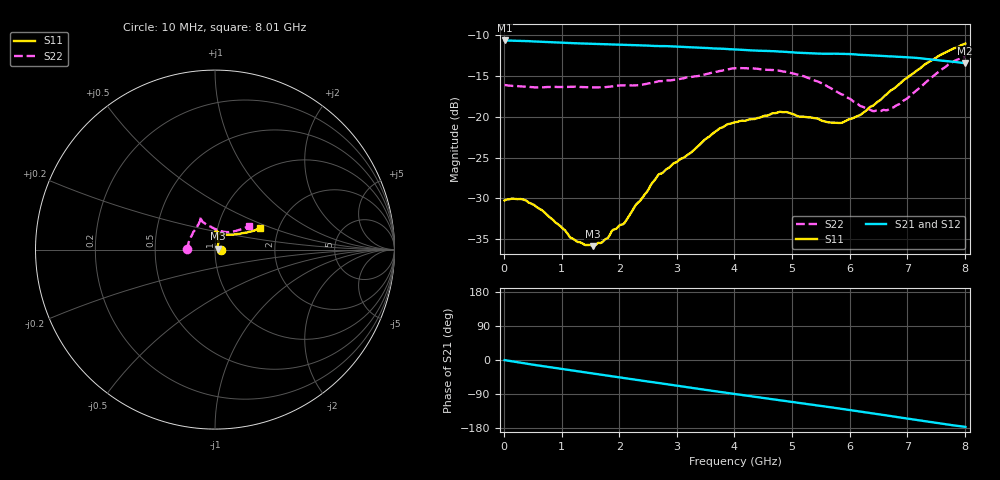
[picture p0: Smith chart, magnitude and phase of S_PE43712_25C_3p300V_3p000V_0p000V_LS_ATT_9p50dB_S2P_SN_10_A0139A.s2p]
! DEVICE ID: PE43712
! File Path: z:\PE43713\PE43713_CHAR_NOM_04292014\AMB\3p300\LS_ATT_9p50dB\PE43713_AMB_3p300V_3p000V_0p000V_LS_ATT_9p50dB_S2P_SN_10_A0139A.s2p
! Serial: 10
! Lot: A0139A
! Temp: 25C
! VDD: 3.300
! VSS: 0.000
! Control_Hi: 3.000
! Control_Lo: 0.000
! Attenuation Step: 9.50dB
! Port 1: RF1
! Port 2: RF2
! ThroughPath:1-2
! IDD: 0.0001469591
! ISS: -2.49e-008
#  Hz  S  RI  R  50
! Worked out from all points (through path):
!   801 points, 10 MHz to 8.01 GHz, reference 50 ohm
!   highest |S21| = -10.66 dB at 10 MHz (marker M1); lowest = -13.4 dB at 8 GHz (marker M2)
!   group delay of S21, straight-line fit = 60.6 ps
!   lowest |S11| = -35.9 dB at 1.54 GHz (marker M3), VSWR 1.03, Z = 51.6 + j0.514 ohm
!   |S11| at or under -10 dB: start of sweep to end of sweep
!   |S22| runs from -19.3 to -12.7 dB; largest |S21 - S12| = 0.0011
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1e7  0.0307 0.000143  0.2932 -0.00153  0.2933 -0.00148  -0.1564 0.000949
3e8  0.0311 -0.00359  0.2886 -0.0381  0.2886 -0.0381  -0.1526 0.0151
5e8  0.0287 -0.0048  0.2827 -0.0616  0.2827 -0.0616  -0.1498 0.0238
1.17e9  0.0181 -0.000596  0.2505 -0.1303  0.2505 -0.1305  -0.1422 0.0552
1.35e9  0.0168 0.00151  0.2398 -0.1467  0.2398 -0.1467  -0.1386 0.0623
1.54e9  0.0153 0.00498  0.2273 -0.1629  0.2273 -0.1629  -0.133 0.0717
1.71e9  0.0147 0.00871  0.2154 -0.1765  0.2154 -0.1765  -0.1289 0.0795
2.09e9  0.0139 0.0175  0.1857 -0.2041  0.1857 -0.204  -0.1211 0.0977
2.68e9  0.0192 0.0397  0.1329 -0.2361  0.1328 -0.2361  -0.0985 0.1322
3.72e9  0.0136 0.0826  0.0297 -0.2596  0.0295 -0.2596  -0.0825 0.1707
4.01e9  0.0104 0.0919  0.000998 -0.2584  0.000956 -0.2584  -0.085 0.179
4.79e9  0.00542 0.1071  -0.0707 -0.2404  -0.0708 -0.2407  -0.0802 0.1734
5.35e9  0.0159 0.0971  -0.1152 -0.216  -0.1152 -0.2159  -0.0693 0.1549
5.88e9  0.0387 0.0837  -0.154 -0.1874  -0.1537 -0.1874  -0.0331 0.1323
6.18e9  0.0606 0.0824  -0.1727 -0.166  -0.1724 -0.166  -0.0045 0.1166
6.39e9  0.0805 0.0837  -0.1837 -0.1504  -0.1834 -0.1503  0.0172 0.1074
6.68e9  0.1128 0.0851  -0.1971 -0.1268  -0.1968 -0.1269  0.0508 0.0985
7e9  0.1476 0.0905  -0.2088 -0.0994  -0.2085 -0.0993  0.0846 0.098
7.35e9  0.1895 0.0992  -0.2152 -0.0672  -0.215 -0.0672  0.126 0.1075
7.72e9  0.2283 0.1102  -0.2156 -0.035  -0.2155 -0.0352  0.1692 0.1228
8e9  0.2518 0.1213  -0.2124 -0.0133  -0.2121 -0.0137  0.1907 0.1327
8.01e9  0.2524 0.1221  -0.2124 -0.0127  -0.2121 -0.0132  0.1913 0.133
